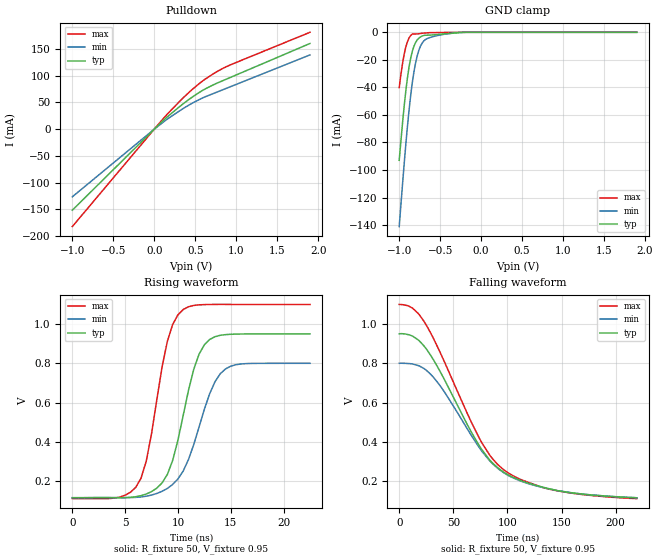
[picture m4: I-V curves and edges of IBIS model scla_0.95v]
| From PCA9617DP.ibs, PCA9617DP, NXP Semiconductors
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[Model]   scla_0.95v
Model_type Open_drain
Vref=9.500E-01
Rref=1.350E+03
Cref=5.000E-11
Vmeas=4.250E-01
C_comp   9.000E-13   8.790E-13   9.210E-13
[Voltage Range]   9.500E-01   8.000E-01   1.100E+00
[POWER Clamp Reference]   9.500E-01   8.000E-01   1.100E+00
[GND Clamp Reference]   0.000E+00   0.000E+00   0.000E+00
[Pullup Reference]   9.500E-01   8.000E-01   1.100E+00
[Pulldown Reference]   0.000E+00   0.000E+00   0.000E+00
[Temperature Range]   25   85   -40
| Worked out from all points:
|   slope of the pulldown table from 0 to 0.142 V, typ, clamps not added: 6.87 ohm
|   GND clamp passes 1 mA (typ) near -0.42 V on its own axis
|   rising waveform, R_fixture 50, V_fixture 0.95: 20-80 % time 2.25ns typ, 2.65ns min, 1.93ns max; typ from 0.115 V to 0.95 V
|   falling waveform, R_fixture 50, V_fixture 0.95: 20-80 % time 52.9ns typ, 53.5ns min, 53.3ns max; typ from 0.95 V to 0.115 V
[GND Clamp]
-1V       -92.92mA   -141mA     -40.15mA
-960mV    -66.21mA   -110.7mA   -22.9mA
-920mV    -42.87mA   -81.83mA   -10.8mA
-880mV    -25.23mA   -56.59mA   -4.143mA
-840mV    -13.8mA    -36.49mA   -1.263mA
-800mV    -7.405mA   -22.14mA   -1.234mA
-760mV    -4.222mA   -13.02mA   -1.081mA
-720mV    -2.709mA   -7.844mA   -694.3uA
-680mV    -2.13mA    -5.24mA    -486.3uA
-540mV    -1.616mA   -2.438mA   -205.2uA
-260mV    -205.4uA   -87.9uA    -30.71uA
1.9V      0A         0A         0A
[Pulldown]
-1V       -151.8mA   -126.7mA   -182.5mA
140mV     20.4mA     16.69mA    24.94mA
360mV     48.38mA    39.38mA    59.74mA
520mV     65.97mA    53.29mA    81.76mA
720mV     83.02mA    66.7mA     103.6mA
900mV     95.06mA    77.75mA    118.5mA
1.9V      160.6mA    139.2mA    181.6mA
[Rising Waveform]
R_fixture = 50
V_fixture = 0.95
V_fixture_min = 0.8
V_fixture_max = 1.1
0s        114.6mV    114.6mV    110.1mV
4ns       114.8mV    115mV      112.7mV
6ns       119.5mV    116.3mV    167mV
7ns       133.4mV    122.3mV    301.3mV
9ns       233.6mV    162.1mV    912.8mV
10.5ns    534.9mV    251.1mV    1.074V
12ns      846.7mV    475.5mV    1.098V
13.5ns    935.6mV    705.3mV    1.1V
14.5ns    946.3mV    771.3mV    1.1V
22.5ns    950mV      800mV      1.1V
[Falling Waveform]
R_fixture = 50
V_fixture = 0.95
V_fixture_min = 0.8
V_fixture_max = 1.1
0s        950mV      800mV      1.1V
12.5ns    938mV      796.3mV    1.08V
23ns      887.4mV    772.7mV    1.013V
38ns      755.9mV    684mV      852.8mV
74.5ns    375.3mV    366.4mV    413.3mV
85ns      298.9mV    295.1mV    321.9mV
96.5ns    245.4mV    242.6mV    257.7mV
112.5ns   202.1mV    199.5mV    207.3mV
140.5ns   158.2mV    157.7mV    156.1mV
219.5ns   114.6mV    114.6mV    110.1mV
[Ramp]
dV/dt_r   5.0125E-01/2.2900E-09   4.1125E-01/2.6290E-09   5.9393E-01/1.9220E-09
dV/dt_f   5.0125E-01/5.2793E-08   4.1125E-01/5.3430E-08   5.9393E-01/5.3187E-08
R_load = 50
